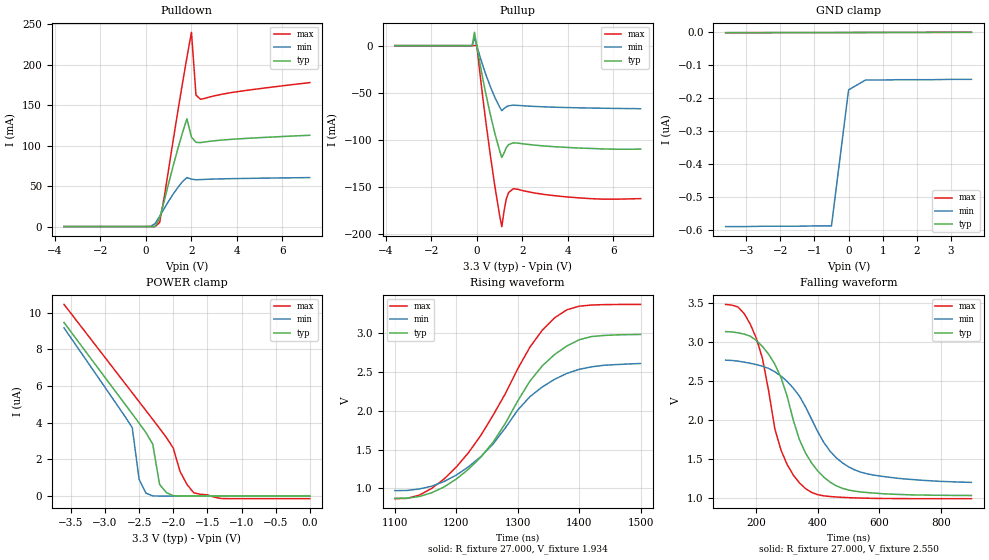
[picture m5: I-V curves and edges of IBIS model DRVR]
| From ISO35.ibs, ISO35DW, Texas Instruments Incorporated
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|   Driver Output / Receiver Input Model
[Model]   DRVR
Model_type   I/O
| Signals   Y,Z
Vinl = 0.9V
Vinh = 2.8V
Vmeas = 1.7V   |Reference voltage for timing measurements
Cref = 50pF   |Timing specification test load capacitance value
Rref = 54   |Note: 54 Ohm load; single-ended configuration
|   Timing specification test load voltage
| variable   typ   min   max
C_comp   28pF   24pF   32pF
|   typ   min   max
[Temperature Range]   25.0   -40   85
[Voltage range]   3.3V   3.0V   3.6V
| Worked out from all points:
|   slope of the pulldown table from 0 to 0.495 V, typ, clamps not added: 101 ohm
|   slope of the pullup table from 0 to 0.495 V, typ, clamps not added: 7.99 ohm
|   rising waveform, R_fixture 27.000, V_fixture 1.934: 20-80 % time 112ns typ, 113ns min, 114ns max; typ from 0.873 V to 2.98 V
|   falling waveform, R_fixture 27.000, V_fixture 2.550: 20-80 % time 119ns typ, 151ns min, 88.8ns max; typ from 3.14 V to 1.03 V
[Pulldown]
|   Voltage   I(typ)   I(min)   I(max)
-3.6V     159.9pA    -3.538nA   187pA
200mV     102.5nA    84.16uA    637.5pA
400mV     125.5uA    3.658mA    2.583uA
600mV     10.13mA    12.54mA    4.944mA
800mV     31.32mA    22.18mA    35.61mA
1.2V      75.16mA    40.21mA    107mA
1.8V      133.2mA    60.51mA    208.6mA
2V        110.4mA    58.58mA    239.9mA
2.2V      104mA      57.81mA    162.4mA
2.4V      103.7mA    57.98mA    157.1mA
3.8V      107.8mA    59.18mA    165.7mA
7.2V      112.7mA    60.46mA    177.8mA
[Pullup]
|   Voltage   I(typ)   I(min)   I(max)
| Note that the[Pullup]voltage table is referenced to Vcc
| and is calculated using Vtable=Vcc - Vmeasured.
-3.6V     10.65uA    9.229uA    12.84uA
-200mV    2.036uA    2.463uA    2.347uA
-100mV    14.15mA    8.567mA    2.306uA
0V        206.6uA    144.9uA    382uA
300mV     -39.21mA   -23.56mA   -61.72mA
600mV     -73.39mA   -43.64mA   -116.8mA
1.1V      -118.5mA   -68.93mA   -191.7mA
1.3V      -108mA     -64.78mA   -162.1mA
1.4V      -104.9mA   -63.71mA   -155.7mA
1.6V      -102.9mA   -63.05mA   -151.6mA
4V        -107.9mA   -65.61mA   -160.4mA
7.2V      -109.6mA   -66.83mA   -162.1mA
[GND_clamp]
|   Voltage  I(typ)   I(min)   I(max)
| Outputs in High Impedance (off)
-3.6V     -974pA     -591nA     -897pA
-500mV    -651pA     -589nA     -575pA
0V        -527pA     -175nA     -523pA
500mV     -357pA     -145nA     -425pA
3.6V      186pA      -143nA     105pA
[POWER_clamp]
|   Voltage  I(typ)   I(min)   I(max)
| Note that the [POWER_clamp] voltage table is referenced to Vcc
| and is calculated using Vtable = Vcc - Vmeasured.
| Outputs in Tri-state.
-3.6V     9.461uA    9.171uA    10.45uA
-2.6V     4.476uA    3.728uA    5.628uA
-2.5V     3.975uA    913.7nA    5.145uA
-2.4V     3.462uA    159.9nA    4.662uA
-2.3V     2.832uA    5.888nA    4.177uA
-2.2V     629.7nA    839.3pA    3.69uA
-2.1V     188.2nA    418.3pA    3.19uA
-2V       18.21nA    442.3pA    2.618uA
-1.9V     1.35nA     417.4pA    1.34uA
-1.7V     446.8pA    389pA      176.4nA
-1.3V     361.5pA    326.9pA    -134nA
0V        132.8pA    105.2pA    -143.4nA
[Ramp]
|   typ   min   max
dV/dt_r   1.27V/113ns   0.96V/115ns   1.50V/114ns
dV/dt_f   1.27V/119ns   0.96V/171ns   1.50V/98ns
R_load = 27ohm | Note: The measurement is on a single-ended configuration
|   with 54ohm line-to-line.
[Rising Waveform]
R_fixture = 27.000
V_fixture = 1.934
V_fixture_min = 1.788
V_fixture_max = 2.122
C_fixture = 0.000
L_fixture = 0.000
|  time   V(typ)   V(min)   V(max)
1.1us     873mV      972.3mV    869mV
1.14us    897mV      994mV      915mV
1.2us     1.121V     1.171V     1.275V
1.24us    1.403V     1.41V      1.682V
1.26us    1.595V     1.573V     1.942V
1.32us    2.38V      2.18V      2.817V
1.36us    2.721V     2.402V     3.192V
1.38us    2.83V      2.478V     3.295V
1.42us    2.951V     2.562V     3.356V
1.5us     2.978V     2.605V     3.364V
[Falling Waveform]
R_fixture = 27.000
V_fixture = 2.550
V_fixture_min = 2.276
V_fixture_max = 2.843
C_fixture = 0.000
L_fixture = 0.000
|  time   V(typ)   V(min)   V(max)
100ns     3.137V     2.769V     3.487V
180ns     3.078V     2.729V     3.234V
220ns     2.944V     2.691V     2.788V
240ns     2.846V     2.663V     2.372V
260ns     2.717V     2.619V     1.887V
280ns     2.547V     2.565V     1.612V
360ns     1.573V     2.167V     1.116V
440ns     1.199V     1.596V     1.014V
520ns     1.083V     1.357V     996.2mV
900ns     1.027V     1.196V     986.2mV
